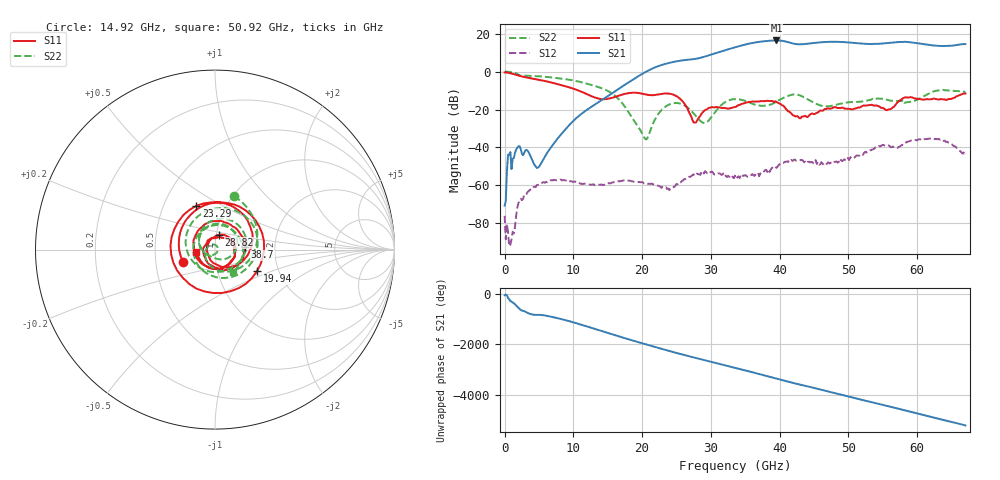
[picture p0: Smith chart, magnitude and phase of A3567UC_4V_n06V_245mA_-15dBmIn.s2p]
! MARKI MICROWAVE INC.
! Date:  4/20/2021
! Model Number:  A-3567UC
! Description:  2-port Small Signal S-parameter data for A-3567UC
! Frequency Range:  10 MHz to 67 GHz
! Port Configuration:  PORT 1: Input
!  PORT 2: Output
! Bias Condition: Vd = +4V, Vg = -0.6V, Id = 245mA
! A-3567UC s2p files are only valid for small signal conditions (below -10 dBm input power)
# Hz S  dB  R 50
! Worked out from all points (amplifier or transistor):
!   401 points, 10 MHz to 67 GHz, reference 50 ohm
!   highest |S21| = 16.5 dB at 39.53 GHz (marker M1)
!   |S21| within 3 dB of that: 34.1 GHz to end of sweep
!   unconditionally stable (mu >= 1): 178.6 MHz to end of sweep
!   at 11.06 GHz: K = 3991.78, MAG = -20.7 dB, |S12| = -59.2 dB
!   at 33.51 GHz: K = 60.34, MAG = 13.1 dB, |S12| = -54.9 dB
!   at 67 GHz: K = 12.01, MAG = 15.3 dB, |S12| = -43.5 dB
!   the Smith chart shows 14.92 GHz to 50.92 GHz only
!   S11 on the Smith chart (normalised r, x): 14.92 GHz: 0.69, -0.10; 19.94 GHz: 1.54, -0.40; 23.29 GHz: 0.73, +0.38; 28.82 GHz: 1.03, +0.17; 38.7 GHz: 1.40, +0.04; 50.92 GHz: 0.81, -0.02
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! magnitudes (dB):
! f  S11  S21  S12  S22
! 10 MHz  -0.4  -70.8  -76.1  0.0
! 679.9 MHz  -0.7  -43.9  -92.2  -0.1
! 1.852 GHz  -1.9  -40.2  -71.9  -1.2
! 4.867 GHz  -4.2  -50.7  -59.8  -2.4
! 11.23 GHz  -10.7  -22.1  -59.2  -5.6
! 14.92 GHz  -14.4  -13.2  -59.4  -10.0
! 19.94 GHz  -11.6  -1.3  -58.3  -32.3
! 20.78 GHz  -12.2  0.4  -59.2  -35.0
! 22.45 GHz  -12.0  3.1  -60.4  -21.9
! 23.29 GHz  -11.5  4.0  -61.2  -18.7
! 25.63 GHz  -14.7  5.9  -58.4  -17.0
! 27.64 GHz  -26.8  6.7  -55.0  -22.7
! 28.82 GHz  -21.4  7.6  -52.6  -26.9
! 33.51 GHz  -18.6  12.9  -54.9  -14.5
! 38.7 GHz  -15.4  16.4  -51.8  -17.3
! 39.53 GHz  -15.9  16.5  -50.8  -15.9
! 44.73 GHz  -22.1  15.1  -47.8  -15.9
! 50.92 GHz  -19.5  15.1  -45.3  -16.0
! 55.95 GHz  -19.9  15.2  -39.1  -15.2
! 58.29 GHz  -13.5  15.8  -37.8  -16.2
! 63.15 GHz  -14.7  13.6  -35.5  -9.9
! 67 GHz  -11.5  14.6  -43.5  -10.7
